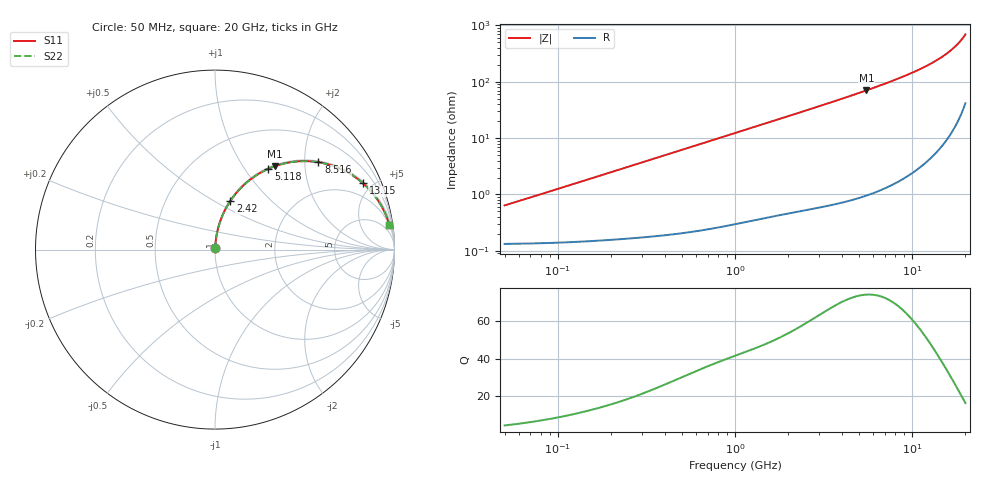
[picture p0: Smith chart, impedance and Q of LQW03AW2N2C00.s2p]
!Murata Part Number: LQW03AW2N2C00
!These Parameters are Measured in Series Mode Connection
!  o--[Z]--o
!Port1  Port2
!  o-------o
!Freq. Start=50[MHz] Stop=20[GHz], 401[Steps]
# Hz S RI R 50
!Freq.(Hz) S11(Real) S11(Imag) S21(Real) S21(Imag) S12(Real) S12(Imag) S22(Real) S22(Imag)
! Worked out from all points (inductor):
!   401 points, 50 MHz to 20 GHz, reference 50 ohm
!   read as one part in series: L = 1.99 nH near 51.52 MHz
!   highest Q = 73.7 at 5.516 GHz (marker M1), where L = 2.03 nH
!   S11 on the Smith chart (normalised r, x): 50 MHz: 1.00, +0.01; 2.42 GHz: 1.01, +0.59; 5.118 GHz: 1.02, +1.29; 8.516 GHz: 1.03, +2.34; 13.15 GHz: 1.10, +4.42; 20 GHz: 2, +14
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5e7  0.00136 0.00625  0.9986 -0.00625  0.9986 -0.00625  0.00136 0.00625
1.364002e8  0.00174 0.017  0.9983 -0.017  0.9983 -0.017  0.00174 0.017
3.721004e8  0.00394 0.0458  0.9961 -0.0458  0.9961 -0.0458  0.00394 0.0458
6.285508e8  0.0082 0.0767  0.9918 -0.0767  0.9918 -0.0767  0.0082 0.0767
1e9  0.0177 0.1204  0.9823 -0.1204  0.9823 -0.1204  0.0177 0.1204
1.639343e9  0.0424 0.1917  0.9576 -0.1917  0.9576 -0.1917  0.0424 0.1917
2.419936e9  0.0851 0.2705  0.9149 -0.2705  0.9149 -0.2705  0.0851 0.2705
2.728004e9  0.1051 0.2986  0.8949 -0.2986  0.8949 -0.2986  0.1051 0.2986
3.792786e9  0.1851 0.3812  0.8149 -0.3812  0.8149 -0.3812  0.1851 0.3812
5.117541e9  0.2979 0.4506  0.7021 -0.4506  0.7021 -0.4506  0.2979 0.4506
5.515528e9  0.3327 0.4644  0.6673 -0.4644  0.6673 -0.4644  0.3327 0.4644
6.406762e9  0.4097 0.485  0.5903 -0.485  0.5903 -0.485  0.4097 0.485
7.442007e9  0.495 0.493  0.505 -0.493  0.505 -0.493  0.495 0.493
8.516016e9  0.576 0.4868  0.424 -0.4868  0.424 -0.4868  0.576 0.4868
1.050288e10  0.7025 0.4487  0.2975 -0.4487  0.2975 -0.4487  0.7025 0.4487
1.183995e10  0.7705 0.411  0.2295 -0.411  0.2295 -0.411  0.7705 0.411
1.314879e10  0.825 0.3692  0.175 -0.3692  0.175 -0.3692  0.825 0.3692
1.482269e10  0.8797 0.3124  0.1203 -0.3124  0.1203 -0.3124  0.8797 0.3124
1.646126e10  0.9197 0.256  0.0803 -0.256  0.0803 -0.256  0.9197 0.256
1.800918e10  0.9473 0.2037  0.0527 -0.2037  0.0527 -0.2037  0.9473 0.2037
1.940974e10  0.9655 0.1579  0.0345 -0.1579  0.0345 -0.1579  0.9655 0.1579
2e10  0.9714 0.1391  0.0286 -0.1391  0.0286 -0.1391  0.9714 0.1391
